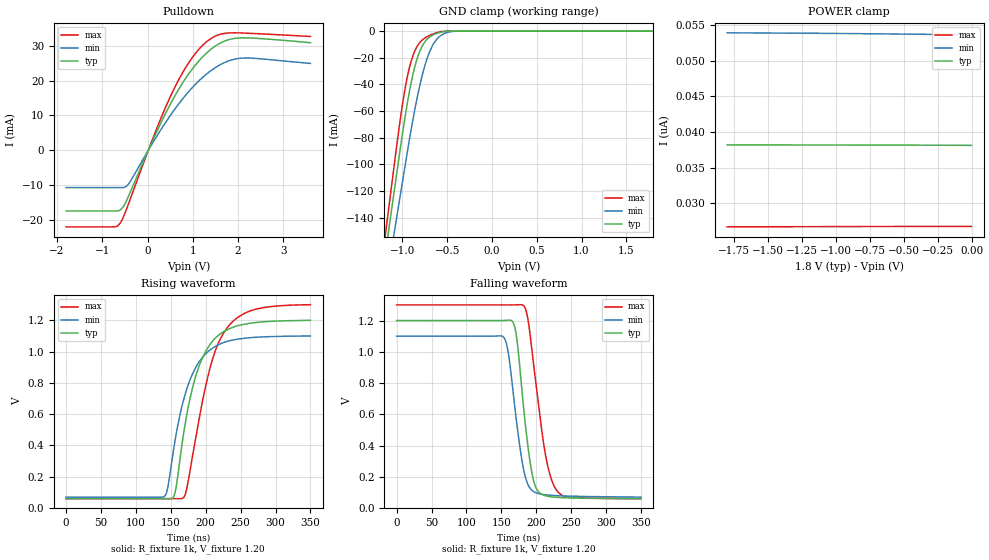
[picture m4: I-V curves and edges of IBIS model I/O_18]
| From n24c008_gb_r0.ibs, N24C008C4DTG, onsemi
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|//////////////////////////////////////////////////////////////////////////////
|//////////////////////////////////////////////////////////////////////////////
[Model] I/O_18
Model_type I/O_open_drain
Vinh =  0.96
Vinl =  0.24
Vmeas = 0.60
Vref = 1.20
Rref = 1000
Cref = 100pF
|  variable   typ   min   max
C_comp   4.60pF   4.60pF   4.60pF
|//////////////////////////////////////////////////////////////////////////////
[Temperature Range]   25   125   -40
|//////////////////////////////////////////////////////////////////////////////
[Voltage Range]   1.80V   1.65V   1.95V
|//////////////////////////////////////////////////////////////////////////////
[Pulldown Reference]   0V   0V   0V
|//////////////////////////////////////////////////////////////////////////////
[POWER Clamp Reference] 1.80V   1.65V   1.95V
|////////////////////////////////////////////////////////////////////////
[GND Clamp Reference]   0V   0V   0V
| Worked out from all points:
|   slope of the pulldown table from 0 to 0.27 V, typ, clamps not added: 35.1 ohm
|   GND clamp passes 1 mA (typ) near -0.58 V on its own axis
|   falling waveform, R_fixture 1k, V_fixture 1.20: 20-80 % time 16.5ns typ, 17.7ns min, 21.9ns max; typ from 1.2 V to 0.06 V
|   rising waveform, R_fixture 1k, V_fixture 1.20: 20-80 % time 34.2ns typ, 34.4ns min, 37.8ns max; typ from 0.06 V to 1.2 V
|//////////////////////////////////////////////////////////////////////////////
[Pulldown]
|   Voltage   I(typ)   I(min)   I(max)
-1.8V     -17.51mA   -10.77mA   -22.06mA
-730mV    -17.51mA   -10.77mA   -22.05mA
-600mV    -17.19mA   -10.77mA   -20.91mA
-480mV    -14.99mA   -10.53mA   -17.53mA
-390mV    -12.36mA   -9.181mA   -14.38mA
200mV     5.189mA    3.891mA    6.07mA
560mV     14.53mA    10.99mA    16.89mA
960mV     22.8mA     17.54mA    26.05mA
1.32V     28.08mA    22.02mA    31.3mA
1.68V     31.21mA    25.03mA    33.49mA
2.04V     32.24mA    26.39mA    33.68mA
3.6V      30.87mA    24.91mA    32.66mA
|//////////////////////////////////////////////////////////////////////////////
[GND Clamp]
|   Voltage   I(typ)   I(min)   I(max)
-1.8V     -456mA     -444.8mA   -474.7mA
-1.18V    -162.7mA   -188.5mA   -148.1mA
-1.14V    -143.8mA   -171.9mA   -127mA
-1.08V    -115.4mA   -147.1mA   -95.39mA
-1V       -77.93mA   -114mA     -55.94mA
-940mV    -52.69mA   -89.26mA   -33.21mA
-900mV    -38.34mA   -73.47mA   -22.4mA
-840mV    -21.88mA   -52.02mA   -12.13mA
-740mV    -7.398mA   -24.13mA   -4.871mA
-620mV    -1.831mA   -6.572mA   -1.298mA
-460mV    -63.11uA   -481.9uA   -13.32uA
1.8V      38.12nA    53.68nA    26.72nA
|//////////////////////////////////////////////////////////////////////////////
[POWER Clamp]
|   Voltage   I(typ)   I(min)   I(max)
-1.8V     38.19nA    53.92nA    26.67nA
-1.26V    38.17nA    53.87nA    26.69nA
-1.14V    38.17nA    53.86nA    26.7nA
-1.08V    38.17nA    53.85nA    26.7nA
-900mV    38.16nA    53.82nA    26.71nA
-660mV    38.15nA    53.78nA    26.72nA
-480mV    38.15nA    53.74nA    26.73nA
-360mV    38.14nA    53.72nA    26.73nA
-240mV    38.14nA    53.7nA     26.73nA
-120mV    38.13nA    53.68nA    26.73nA
0V        38.12nA    53.65nA    26.73nA
|//////////////////////////////////////////////////////////////////////////////
|//////////////////////////////////////////////////////////////////////////////
[Ramp]
|  variable   typ   min   max
dV/dt_r   1.033E-00/2.500E-10  0.936E-00/2.500E-10  1.092E+00/2.000E-10
dV/dt_f   1.033E-00/1.650E-08  0.936E-00/1.800E-08  1.125E+00/2.250E-08
R_load = 1k
|//////////////////////////////////////////////////////////////////////////////
|//////////////////////////////////////////////////////////////////////////////
[Falling Waveform]
R_fixture = 1k
V_fixture = 1.20
V_fixture_min = 1.10
V_fixture_max = 1.30
C_fixture = 0p
|   time   V(typ)   V(min)   V(max)
0s        1.2V       1.1V       1.3V
153ns     1.2V       1.094V     1.3V
160.5ns   1.202V     977.7mV    1.3V
169.5ns   1.153V     639.3mV    1.3V
181.5ns   659.7mV    256mV      1.297V
187.5ns   416.9mV    156.5mV    1.224V
198ns     147.8mV    101.3mV    853.2mV
213ns     79.09mV    85.21mV    346.1mV
228ns     69.09mV    79.74mV    121.4mV
350ns     60mV       70mV       60mV
|//////////////////////////////////////////////////////////////////////////////
[Rising Waveform]
R_fixture = 1k
V_fixture = 1.20
V_fixture_min = 1.10
V_fixture_max = 1.30
C_fixture = 0p
|   time   V(typ)   V(min)   V(max)
0s        60mV       70mV       60mV
141ns     60mV       74.28mV    60mV
145.5ns   60mV       127.4mV    60mV
156ns     97.12mV    429.4mV    60mV
168ns     466.5mV    686mV      65.38mV
192ns     924.4mV    943.7mV    603.8mV
210ns     1.068V     1.023V     954.7mV
228ns     1.133V     1.061V     1.135V
267ns     1.183V     1.09V      1.265V
350ns     1.2V       1.1V       1.3V
